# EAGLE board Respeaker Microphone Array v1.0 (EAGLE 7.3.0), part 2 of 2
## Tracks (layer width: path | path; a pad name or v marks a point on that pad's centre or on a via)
24MHZ  (via drill 0.25 pad 0.51)
  Top 0.203: U1.125 30.04,56.79 v29.96,56.87
  Top 0.305: v29.96,56.88 v29.96,56.87 30.15,57.07 R1.2
  Bottom 0.305: 24M.T 29.33,57.5 v29.96,56.87
24MHZ_8960  (via drill 0.25 pad 0.51)
  Top 0.254: U6.11 37.08,26.89 v37.07,26.9
  Top 0.406: R19.2 36.96,26.77 37.08,26.89
  Bottom 0.406: v37.07,26.9 37.07,27.28 24M_1.T
$123  (via drill 0.25 pad 0.51)
  Top 0.254: U6.29 43.6,26.39 v43.67,26.45
  Top 0.406: C90.1 49.51,21.82 48.5,22.83 v48.5,22.96
  Bottom 0.406: v43.67,26.45 43.8,26.58 44.43,26.58 44.94,26.07 44.94,24.1 46.08,22.96 v48.5,22.96
$124  (via drill 0.25 pad 0.51)
  Top 0.254: U6.31 43.63,27.39 v43.67,27.34
  Top 0.406: C91.1 47.86,21.82 | C91.1 47.48,21.82 | 46.47,21.69 46.59,21.56 46.97,21.56 47.1,21.69 C91.1 | v47.86,23.6 47.86,22.58 C91.1
  Bottom 0.406: v43.67,27.34 43.8,27.22 44.88,27.22 45.58,26.52 45.58,24.36 46.34,23.6 v47.86,23.6
_I2S_BCLK  (via drill 0.25 pad 0.51)
  Top 0.152: U6.12 37.44,26.39 36.94,25.88 v36.69,25.88 | v20.81,49.89 C83.1 R33.1
  Bottom 0.152: v36.69,25.88 35.92,26.64 35.92,31.6 34.65,32.87 34.65,39.47 35.42,40.23 35.42,41.76 33.38,43.79 30.21,43.79 25.38,38.96 20.94,38.96 19.03,40.87 19.03,48.11 v20.81,49.89
_I2S_DAC_DATA  (via drill 0.25 pad 0.51)
  Top 0.152: U6.14 37.59,25.39 37.19,24.99 v35.8,24.99 | v18.02,45.44 C80.1 R41.1
  Bottom 0.152: v35.8,24.99 35.16,25.63 35.16,31.34 33.89,32.61 33.89,39.73 34.65,40.49 34.65,41.5 33.13,43.03 30.59,43.03 25.76,38.2 20.69,38.2 18.02,40.87 v18.02,45.44
_I2S_LRCK  (via drill 0.25 pad 0.51)
  Top 0.152: U6.13 37.58,25.89 37.07,25.37 36.31,25.37 v35.8,25.88 | v18.53,47.6 C82.1 R40.1
  Bottom 0.152: v35.8,25.88 35.54,26.14 35.54,31.47 34.27,32.74 34.27,39.6 35.04,40.36 35.04,41.63 33.26,43.41 30.46,43.41 25.64,38.58 20.81,38.58 18.53,40.87 v18.53,47.6
AGND  (via drill 0.25 pad 0.51)
  Top 0.152: v39.48,27.03 v40.5,27.03 v41.51,27.03 | v39.48,25.25 v40.5,25.25 v41.51,25.25
  Top 0.203: SW1.3 43.58,16.07 43.29,16.36 v43.29,16.61 | SW1.7 44.36,14.33 44.43,14.26 44.62,14.26 | 44.62,14.26 45.13,14.26 v45.2,14.33 44.94,14.33 44.76,14.51 SW1.8 44.76,14.4 44.62,14.26
  Top 0.254: C4.1 44.54,26.37 44.06,25.89 U6.28 40.75,25.89 U6.33
  Top 0.305: R3.1 47.74,16.61 | 46.66,13.75 46.72,13.69 | D2.2 42.21,14 42.02,13.82 | D1.2 43.09,16.81 v43.29,16.61
  Top 0.356: R3.1 46.74,16.59 46.72,16.61 C92.1 46.72,16.76 45.12,18.37 C79.1
  Top 0.406: C89.1 45.55,27.56 v45.7,27.41
  Top 0.508: C89.1 45.55,28.45 | C71.1 45.7,29.18 | 45.58,32.61 U7.1 44.05,32.36 v43.93,32.49 | J9.5 37.09,0.97 36.81,1.24 36.81,1.75 | 36.81,1.75 R32.2 | J9.6 37.31,3.27 36.81,2.77 36.81,1.75
  Top 1.016: v50.07,28.76 48.45,28.76 v46.72,27.03 | 50.23,28.76 v50.07,28.76 | J3.14 v50.7,28.76 50.61,28.76 | 50.58,28.76 v50.07,28.76 | v50.07,28.76 50.02,28.8 | 50.61,28.76 50.58,28.76 | 50.58,28.76 49.89,29.44 | 50.61,28.76 50.02,28.17
  Bottom 1.016: J3.14 v50.07,28.76
  other vias: 40.24,0.99 44.05,2.01 44.05,5.18 46.72,12.93 42.53,13.44 42.53,17.37 46.59,26.14 40.5,26.14 39.48,26.14 41.51,26.14 40.12,29.95 41.39,29.95 44.43,11.28 40.37,7.72 43.42,6.96 40.75,5.18 38.08,2.13 38.21,9.63 38.21,15.98 38.21,17.37 39.48,17.37 40.75,17.37 46.47,11.28 45.45,11.28 42.4,32.49 44.81,30.84 44.81,29.31 38.85,2.13 39.61,2.13 43.54,8.74 41.64,10.01 43.67,10.01 42.53,11.53 44.05,12.55 41.64,13.06 48.37,30.84 49.64,30.84 49.64,31.85 48.37,31.85 41.39,31.22 38.21,14.71 38.21,13.44 38.21,12.17 48.24,26.01 48.37,29.31 48.37,12.93 49.01,14.33 50.91,14.33 48.37,11.66 46.59,6.58 46.72,3.91 49.18,26.03 47.35,26.01
  pour Top (isolate 0.254, rank 2): 45.7,-0.53 36.31,-0.53 36.31,4.17 37.07,4.93 37.19,16.98 37.18,18.18 arc-90 38.65,19.66 39.93,19.66 arc45 40.5,20.23 40.5,23.85 39.74,23.85 38.92,24.67 38.92,30.1 41.58,32.75 47.74,32.74 50.76,32.74 arc-90 52.31,31.19 52.31,28.8 52.32,24.8 52.31,24.61 52.31,24.49 52.31,13.44 52.32,13.45 52.31,13.06 52.31,11.15 arc-90 50.77,9.61 50.67,9.61 50.66,9.63 50.15,9.61 48.88,9.63 48.05,9.63 arc90 46.85,8.43 46.85,0.61
  pour PWR (isolate 0.254): 46.34,-0.53 37.96,-0.53 37.58,-0.15 37.58,16.96 38.11,17.5 49.95,17.5 52.31,15.14 52.31,12.8 47.71,10.9 47.59,10.9 46.85,10.16 46.85,-0.03
  pour PWR (isolate 0.254): 41.61,32.76 49.59,32.76 50.28,32.07 50.28,26.57 49.46,25.76 43.54,25.76 42.27,24.48 39.57,24.48 39.13,24.91 39.13,30.28
  pour Top (isolate 0.254, no thermals): 39.1,-0.03 36.69,-0.03 36.43,0.23 36.43,3.4 37.07,4.04 39.86,4.04 40.12,3.78 40.12,0.1 39.99,-0.03
AUX_SEL  (via drill 0.25 pad 0.51)
  Top 0.203: SW1.6 43.58,14.87 43.42,14.71 v43.42,13.56 R20.2 | J3.1 60.42,40.76 v60.44,40.74
  Bottom 0.203: v43.42,13.56 56.75,13.56 62.34,19.15 62.34,39.34 60.93,40.76 60.45,40.76 v60.44,40.74 60.42,40.76 J3.1
AVDD  (via drill 0.25 pad 0.51)
  Top 0.203: SW1.1 44.76,16.68 v44.94,16.87
  Top 0.254: U6.32 43.39,27.89 43.54,28.04 43.93,28.04
  Top 0.406: C89.2 v44.05,28.04 43.93,28.04 | U7.2 47.35,30.96 C68.2 C71.2 47.23,29.18 46.59,28.55 v46.34,28.55 | C79.2 45.07,16.99 v44.94,16.87 | R20.1 45.04,12.83 v45.07,12.8
  PWR 0.406: v45.07,12.8 44.56,13.31 44.56,16.48 v44.94,16.87 50.53,16.87 v52.82,19.15
  Bottom 0.406: v46.34,28.55 46.34,29.18 TP4.T | v46.34,28.55 45.83,28.55 | 45.83,28.55 44.56,28.55 v44.05,28.04 | v46.34,28.55 47.1,28.55 | 47.1,28.55 47.61,28.55 50.66,25.5 50.66,20.42 51.93,19.15 v52.82,19.15 | 45.83,28.55 46.47,29.18 | 47.1,28.55 46.59,29.06
CENTRAL_LED  (via drill 0.25 pad 0.51)
  Top 0.152: R34.2 33.52,31.09 v33.52,30.59 v33.51,30.58 | U1.32 33.15,41.78 v33.26,41.88 | J3.4 50.83,38.76 v50.28,38.2
  Top 0.305: J3.4 55.44,38.76 v55.48,38.71
  PWR 0.152: v33.51,30.58 33.64,30.45 38.46,30.45 41.39,33.38 45.45,33.38 v50.28,38.2
  Bottom 0.152: v33.51,30.58 33.51,39.85 34.27,40.61 34.27,41.38 33.77,41.88 v33.26,41.88
  Bottom 0.305: J3.4 55.44,38.76 v55.48,38.71
DEBUG_USBDM_N  (via drill 0.25 pad 0.51)
  Top 0.203: J1.2 27.56,6.04 27.69,6.17 27.69,6.83 27.23,7.3 D7.1 27.23,7.54 27.67,7.98 27.67,9.5 v27.54,9.63 27.67,9.75 27.67,10.52 28.18,11.02 31.86,11.02 32.24,11.4 32.24,12.29 31.99,12.55 31.59,12.55 R38.2
  Bottom 0.152: v27.54,9.63 DM.T
DEBUG_USBDP_P  (via drill 0.25 pad 0.51)
  Top 0.203: D8.1 28.49,7.54 | D8.1 28.49,7.49 28.05,7.92 28.05,9.37 v28.3,9.63 28.05,9.88 28.05,10.39 28.3,10.64 32.11,10.64 32.62,11.15 32.62,12.42 32.11,12.93 31.69,12.93 R4.2 | J1.3 28.21,5.99 28.05,6.15 28.05,6.81 28.49,7.25 D8.1
  Bottom 0.152: v28.3,9.63 DP.T
DOUT5  (via drill 0.25 pad 0.51)
  Top 0.152: SK7.3 51.45,10.16 47.99,6.71 v47.99,6.07 | SK6.1 34.79,7.08 v35.67,6.2
  Bottom 0.152: v35.67,6.2 36.05,5.82 47.74,5.82 v47.99,6.07
GND  (via drill 0.25 pad 0.51, 0.64 pad 1.27)
  Top 0.203: U1.104 38.44,54.81 v38.34,54.71
  Top 0.254: U6.20 40.25,22.43 C69.1 | U6.24 42.25,23.24 v42.53,22.96 | U6.9 37.73,27.89 37.58,28.04 v37.58,28.3 | U3.6 23.14,29.4 22.97,29.57
  Top 0.305: U3.6 24.86,29.4 U3.9 | U3.3 25.34,29.4 25.13,29.18 25.13,29.17 U3.9 | U2.6 22.08,21.57 U2.9 21.07,21.82 v20.94,21.69 | U2.3 22.08,22.07 v22.34,21.82 | U5.2 21.57,30.32 v21.51,30.26 | J1.5 29.51,6.01 29.7,6.2 v29.96,6.2 | D7.2 27.14,8.37 v26.91,8.61 | U10.4 34.41,17.59 v34.22,17.4 | MIC7.8 36.74,33.94 36.94,34.14 v37.19,34.14 | MIC7.2 34.37,34.74 34.58,34.96 MIC7.5 35.85,34.96 36.18,35.28 36.18,35.39 v36.17,35.41 | MIC7.7 36.11,32.56 36.31,32.36 v36.31,32.11 | v25.13,29.12 v25.13,29.13 U3.9 | 22.84,21.82 v22.34,21.82 | U2.1 23.08,21.93 v22.97,21.82 v22.34,21.82 | v33.89,57.38 33.89,57.44 34.65,58.2 v34.65,58.39 | v52.43,42.65 52.29,42.5 U11.4 52.29,40.98 52.18,40.87 | 22.46,37.95 22.33,37.81 U9.4 22.33,36.56 22.72,36.17 | MIC8.2 20.36,61.82 v20.43,61.89 | MIC9.2 3.05,34.64 v3.44,35.03 | MIC10.2 18.07,6.79 v18.07,7.04 | MIC11.2 49.82,5.74 v49.77,5.69 | MIC12.2 67.02,32.84 v66.66,32.49 | MIC13.2 51.93,60.76 v51.93,60.43 | MIC12.8 67.44,35.89 v67.42,35.92 | C109.1 67.1,36.42 v66.98,36.3 | C86.1 42.66,33.76 v42.91,34.01 43.01,33.91 C108.1 44.54,33.91 v44.56,33.88 | MIC10.8 20.35,4.84 20.94,5.44 v21.13,5.44 | MIC7.6 33.34,33.65 v32.94,33.25 | C103.1 33.41,9.9 v33.38,9.88 | U3.1 25.54,28.4 | 25.34,28.4 25.13,28.4 25.11,28.42 | 25.54,28.4 25.54,28.01 25.64,27.91 | 25.54,28.4 25.34,28.4 | 25.34,28.4 25.19,28.55 | v22.84,33.69 22.84,34.03 | 22.84,34.03 C87.1 22.74,34.29 22.84,34.39 | 22.84,34.39 23.35,34.9 | 22.84,34.03 22.84,34.39 | D8.2 28.49,8.41 28.69,8.61 v28.94,8.61
  Top 0.356: v25.32,34.52 27.14,34.52 C85.1
  Top 0.406: v25.13,30.71 25.11,30.69 U3.9 25.11,28.42 25.11,28.32 25.51,27.91 | C69.1 v39.48,22.2 | 18.76,7.11 v18.4,7.47 | 49.33,6.12 v49.26,6.2 | MIC7.2 33.43,34.18 33.38,34.14
  Top 0.508: C5.1 v27.41,38.7 v27.42,38.71 | R22.1 22.2,27.91 v21.95,27.66 | C31.1 39.84,58.37 v40.12,58.65 | C39.1 34.68,58.37 v34.65,58.39 | C52.1 36.92,58.37 v36.94,58.39 | C51.1 v37.96,59.02 v37.96,59.03 | R7.1 19.16,25.89 v19.03,26.01 | v28.18,58.14 28.9,58.14 C32.1 | C66.1 31.58,58.37 v31.61,58.39 | C26.1 32.22,58.37 v32.56,58.71 | X1.2 30.53,61.99 C24.1 | C75.1 33.87,57.4 v33.89,57.38 | C62.1 43.95,23.49 v43.93,23.47 | C74.1 45.8,59 v45.83,59.03 | C1.1 36.43,11.66 v36.31,11.53 | C107.1 35.29,27.91 v34.65,28.55 | C88.1 34.78,29.06 v34.65,29.18 | D9.- 36.82,31.09 v36.94,30.96 | X2.2 34.34,24.93 v34.15,24.74 34,24.59 C2.1 34,23.75 v34.02,23.72 | v26.65,27.53 26.65,26.77 27.14,26.29 C19.1 27.76,26.1 v27.8,26.14 | C64.1 17.7,33.12 v17.37,33.45 | v18.53,29.82 18.14,29.44 Q1.2 17.51,29.82 v17.26,29.82 | SK3.2 6.67,36.22 v6.59,36.3 | C57.1 5.53,29.97 v5.51,29.95 | C35.1 30.85,36.86 v31.16,36.55 | C42.1 31.87,36.62 v31.8,36.55 | C41.1 32.88,37 v32.43,36.55 | C34.1 30.82,37.08 30.84,37.06 | v23.73,44.04 24.11,43.66 C40.1 | C65.1 v16.74,55.22 v16.75,55.22 | C45.1 24.4,53.54 v23.99,53.95 | v23.48,42.84 23.48,42.37 C84.1 | C58.1 21.78,5.13 v21.7,5.05 | R32.1 35.82,2.43 v35.73,2.51 | R32.1 v35.1,1.75 | R32.1 35.82,1.2 v35.73,1.12 | v15.35,17.25 14.11,16 C14.1 13,13.5 v12.94,13.44 | C63.1 19.99,34.2 v19.92,34.26 | C85.1 27.9,34.8 28.5,34.2 v28.5,33.95 28.54,33.91 R11.1 | C20.1 24.34,33.86 25,34.52 v25.32,34.52 | C59.1 54.71,8.36 | 54.71,8.36 54.71,9.01 v54.47,9.25 | 54.71,8.36 54.73,8.33 C110.1 56.35,8.33 v56.37,8.36
  Top 0.61: v42.53,22.96 43.42,22.96 v43.93,23.47
  Bottom 0.305: v37.58,28.3 37.7,28.17 37.7,26.52 37.58,26.39
  other vias: 27.8,23.6 23.54,32.68 23.54,32.04 27.16,25.37 30.72,62.84 40.12,60.43 50.91,58.33 45.7,53.82 46.34,49.89 46.34,49 46.34,47.73 46.34,46.71 46.34,44.93 46.34,42.27 39.93,36.42 38.4,36.55 37.39,36.55 36.12,36.55 35.29,36.49 23.8,39.47 50.28,47.73 23.73,45.69 23.73,46.71 23.73,47.73 23.67,51.09 18.4,9.88 12.81,9.63 8.75,21.31 7.22,31.22 9.76,44.55 33.77,67.41 37.58,62.46 55.48,50.27 59.8,51.54 60.44,54.84 61.45,46.2 63.1,37.69 61.2,22.96 53.45,11.02 47.86,8.36 35.92,9.63 23.73,5.31 30.72,5.94 28.69,24.74 35.04,47.98 37.07,47.98 33,47.98 33,49.89 35.04,49.89 37.07,49.89 37.07,46.08 35.04,46.08 33,46.2 62.98,51.54 9,13.44 25.89,27.91 32.75,1.75 7.1,17.25 39.73,35.6 12.18,49.63 61.2,48.87 28.69,66.14 23.61,64.87 17,62.46 7.73,53.44 15.1,51.54 13.45,43.92 6.46,40.11 3.29,26.14 7.1,26.14 3.29,21.69 50.28,51.54 57.9,53.44 55.36,46.46 57.9,56.62 68.06,28.68 55.36,59.16 22.46,13.06 19.16,13.44 47.74,55.35 27.23,2.13 29.26,2.13 41.39,52.81 37.07,52.81 41.39,47.98 41.39,46.08 41.39,49.89 31.86,54.33 35.04,51.54 44.56,55.98 43.93,58.52 41.26,60.68 25.51,58.39 20.43,19.79 19.16,19.79 17.89,19.79 17.89,19.15 19.16,19.15 20.43,19.15 20.43,17.63 19.16,17.63 17.89,17.63 20.43,21.06 23.61,22.2 23.86,22.77 15.35,13.44 17.89,13.44 32.62,28.04 28.69,23.6 35.29,59.16 36.31,59.16 38.85,60.43 24.24,61.06 10.91,53.44 10.91,57.25 29.96,3.28 26.15,3.28 35.54,7.21 47.74,48.36 14.08,45.82 15.99,43.92 15.99,45.82 9,49.63 5.19,49.63 6.46,44.55 3.29,44.55 3.29,40.11 7.1,21.69 15.35,12.17 19.16,12.17 22.97,36.93 65.52,44.55 67.42,41.38 66.15,38.58 47.74,45.19 25.51,54.71 26.15,56.62 51.55,55.35 66.79,24.23 65.9,19.79 32.5,62.97 24.88,62.33 39.1,20.8 20.43,13.44 34.02,21.69 32.62,21.69 32.62,18.01 28.69,17.25 28.69,15.98 23.22,13.69 21.7,13.44 26.65,38.33 48.88,5.18 54.97,11.15 55.74,11.66 54.34,12.04 57.9,13.82 64.69,17.18 19.03,53.44 30.08,62.2 50.28,40.74 19.54,42.27 60.56,13.06 3.29,31.6 1.19,35.09 4.3,34.77 4.56,33.12 20.68,7.09 19.16,3.66 17.13,60.17 20.81,61 20.18,59.98 51.29,63.22 49.01,62.46 50.02,59.92 66.02,32.36 69.07,35.15 53.2,5.05 50.34,7.72 52.75,7.34 48.37,39.47 50.28,35.66 50.28,39.47 55.36,55.35 55.36,52.17 62.98,47.73 13.45,59.79 14.72,57.63 22.97,7.09 33.89,1.75 47.74,2.64 63.04,14.77 58.4,17.37 61.83,17.63 59.67,15.47 63.29,19.15 63.36,21.69 63.36,25.5 63.36,30.58 60.44,25.5 55.36,43.92 58.53,43.92 52.75,43.92 62.28,42.65 64.18,40.74 46.08,41.63 44.05,41.57 24.49,30.71 55.36,42.65 58.53,42.65 48.5,64.43 22.97,47.6 22.97,49.89 23.73,48.74 17.95,50.52 14.08,60.49 20.68,3.02 35.92,10.2 36.56,22.58 37.45,32.11 44.56,35.92 44.56,34.52 17,24.99 14.84,24.99 15.99,19.15 14.08,19.15 11.16,25.88 13.45,29.95 13.45,31.72 13.45,33.76 13.45,39.85 2.27,28.93 46.85,61.51 45.58,62.14 44.94,65.06 41.07,65.06 50.28,34.39 27.42,17.25 42.91,38.58 35.67,15.98 36.56,17.63 36.31,16.87 13.51,19.85 55.99,18.52 53.45,18.52 32.62,4.29 35.54,4.04 47.61,3.91 33.26,13.69 33,15.98 36.56,20.8 32.11,24.23 19.41,38.58 18.02,39.47 30.84,42.39 31.48,42.39
  pour Top (isolate 0.254, rank 6): -0.52,69.32 70.6,69.32 70.6,-0.53 -0.52,-0.53
  pour GND (isolate 0.254, rank 6, no thermals): -0.52,69.32 70.6,69.32 70.6,-0.53 2.02,-0.53 2.02,-1.17 -0.52,-1.17
  pour Bottom (isolate 0.254, rank 6): -0.52,69.32 70.6,69.32 70.6,-0.53 2.02,-0.53 2.02,-2.44 -0.52,-2.44
  pour PWR (isolate 0.254, no thermals): 32.5,50.52 37.58,50.52 37.58,45.44 32.5,45.44
  pour Top (isolate 0.254, rank 2, no thermals): 22.97,6.45 32.5,6.45 32.5,-1.17 22.97,-1.17
  pour Bottom (isolate 0.254, rank 2, no thermals): 22.97,6.45 30.64,6.45 31.1,5.99 31.1,4.67 32.5,3.52 32.5,-1.17 22.97,-1.17
HP_L  (via drill 0.25 pad 0.51)
  Top 0.203: SW1.4 43.17,15.67 v43.05,15.8
  Top 0.356: D1.1 42.47,15.91
  Top 0.406: J3.8 56.13,34.76 v56.24,34.65 | v43.05,15.8 42.93,15.91 D1.1 42.46,15.98 42.4,15.98 41.64,16.74 39.86,16.74 39.61,16.48 L4.1
  Bottom 0.406: J3.8 56.13,34.76 v56.24,34.65 56.24,25.76 58.4,23.6 58.4,19.53 54.67,15.8 v43.05,15.8
HP_R  (via drill 0.25 pad 0.51)
  Top 0.203: SW1.5 43.22,15.27 v43.04,15.09
  Top 0.406: J3.7 57.12,34.76 v57.01,34.65 | v43.04,15.09 42.85,14.9 D2.1 42.21,14.9 41.26,15.85 L3.1
  Bottom 0.406: J3.7 57.12,34.76 v57.01,34.65 57.01,26.01 59.04,23.98 59.04,19.28 54.85,15.09 v43.04,15.09
I2C_SCL  (via drill 0.25 pad 0.51)
  Top 0.152: R37.1 45.75,52.04 v46.21,52.04 46.24,52.07 R15.1 46.72,53.95 45.96,54.71 42.15,54.71 41.13,53.7 36.13,53.7 35.24,54.58 U1.112 | U6.17 38.75,23.5 37.96,22.71 v37.7,22.71
  Bottom 0.152: v46.21,52.04 45.07,50.9 45.07,32.61 42.53,30.07 42.53,24.36 42.15,23.98 38.97,23.98 v37.7,22.71
I2C_SDA  (via drill 0.25 pad 0.51)
  Top 0.152: R36.1 45.75,51.03 v46.21,51.03 46.24,51.06 R16.1 46.72,50.39 47.1,50.01 48.5,50.01 49.01,50.52 49.01,52.55 46.47,55.09 42.02,55.09 41,54.08 36.56,54.08 v36.31,54.33 | U1.113 34.84,54.14 v34.78,54.08 | U6.18 39.25,23.3 38.46,22.52 v38.46,22.07
  Bottom 0.152: v46.21,51.03 45.45,50.27 45.45,32.49 42.91,29.95 42.91,24.23 42.27,23.6 39.46,23.6 38.46,22.6 v38.46,22.07 | v36.31,54.33 35.04,54.33 v34.78,54.08
I2S_BCLK  (via drill 0.25 pad 0.51)
  Top 0.152: U1.15 28.08,48.58 v28.37,48.87 | R33.2 22.91,51.03 v22.97,51.09
  Bottom 0.152: v28.37,48.87 27.99,49.25 22.72,49.25 22.34,49.63 22.34,50.46 v22.97,51.09
I2S_DAC_DATA  (via drill 0.25 pad 0.51)
  Top 0.152: U1.21 29.3,46.18 v29.32,46.2 | R41.2 v22.97,46.46
  Bottom 0.152: v29.32,46.2 29.32,46.84 28.94,47.22 23.48,47.22 22.97,46.71 v22.97,46.46
I2S_LRCK  (via drill 0.25 pad 0.51)
  Top 0.152: U1.18 29.1,47.38 v29.32,47.6 | v22.97,48.74 R40.2
  Bottom 0.152: v29.32,47.6 28.69,48.23 23.48,48.23 v22.97,48.74
LED_DATA  (via drill 0.25 pad 0.51)
  Top 0.152: R44.1 38.82,63.83 v38.72,63.73 | SK0.3 34.17,62.18 v34.27,62.08
  Bottom 0.152: v38.72,63.73 35.92,63.73 v34.27,62.08
LED_DATA_IN  (via drill 0.25 pad 0.51)
  Top 0.152: R45.2 43.93,64.39 v43.93,65.13 43.8,65.25 42.02,65.25 41.77,65 U13.2 | R47.2 24.39,42.62 23.58,43.43 22.99,43.43 | C77.1 22.84,43.43 | 22.84,43.43 22.99,43.43 | 22.84,43.28 v22.84,43.03 22.46,43.41 | 22.84,43.28 22.84,43.43 | 22.99,43.43 22.84,43.28
  Top 0.254: 22.46,43.41 22.65,43.41 22.78,43.28
  PWR 0.152: v22.84,43.03 22.46,43.41 22.46,51.66 v24.88,54.08
  Bottom 0.152: v24.88,54.08 30.08,54.08 31.61,55.6 40.12,55.6 41.77,57.25 41.77,62.97 v43.93,65.13
MCLK  (via drill 0.25 pad 0.51)
  Top 0.152: U1.63 40.84,39.64 42.15,38.33 42.15,37.69 42.4,37.44 U8.2 v43.54,37.44 | R50.1 26.86,35.77 C85.2 30.49,35.77 v30.59,35.66
  PWR 0.152: v43.54,37.44 43.04,36.93 39.61,36.93 38.59,35.92 30.84,35.92 v30.59,35.66
MCLK_TILE1  (via drill 0.25 pad 0.51)
  Top 0.152: U1.20 28.56,46.58 v28.69,46.71 | C84.2 23.9,41.34 v23.92,41.31 24.11,41.5 R49.1
  Bottom 0.152: v28.69,46.71 28.05,46.08 28.05,45.82 29.13,44.74 29.13,44.49 28.88,44.23 28.62,44.23 27.29,45.57 27.03,45.57 26.78,45.31 26.78,45.06 28.11,43.73 28.11,43.47 27.86,43.22 27.61,43.22 26.15,44.68 25.89,44.68 25.51,44.3 25.26,44.3 25,44.55 24.75,44.55 24.49,44.3 24.49,44.11 24.88,43.73 24.88,43.41 24.62,43.15 24.62,42.9 25.95,41.57 25.95,41.31 25.7,41.06 25.45,41.06 25.19,41.31 v23.92,41.31
MIC_CLK
  Top 0.152: R42.1 42.37,34.88 C108.2 43.42,36.55 | 42.77,36.79 U8.1 43.42,36.79 | 43.42,36.79 43.66,36.79 | R48.2 44.34,36.79 43.72,36.79 43.66,36.79 | 43.42,36.55 43.42,36.79 | 43.42,36.55 43.29,36.68 | 43.66,36.79 43.42,36.55
MIC_CLK0  (via drill 0.25 pad 0.51)
  Top 0.152: MIC7.3 34.1,33.33 33,32.23 v33,32.11 | R29.2 21.32,42.29 C101.2 19.69,43.43 v19.54,43.28
  PWR 0.152: v33,32.11 33,32.36 32.88,32.49 26.53,32.49 21.57,37.44 21.57,38.2 21.32,38.46 20.68,38.46 20.56,38.58 20.56,38.96 20.68,39.09 22.65,39.09 22.78,39.22 22.78,39.6 22.65,39.73 21.57,39.73 21.45,39.85 21.45,40.23 21.57,40.36 22.65,40.36 22.78,40.49 22.78,40.87 22.65,41 21.57,41 19.54,43.03 v19.54,43.28
  Bottom 0.152: MIC_CLK0.T | MIC_CLK0.T 20.56,43.91 | MIC_CLK0.T 20.17,43.91 v19.54,43.28
MIC_CLK1  (via drill 0.25 pad 0.51)
  Top 0.152: MIC8.3 19.69,62.96 19.69,63.37 19.92,63.6 20.81,63.6 21.23,64.02 21.41,64.02 21.64,63.79 21.64,63.67 21.22,63.25 21.22,63.07 21.45,62.84 21.64,62.84 22.02,63.22 22.21,63.22 22.4,63.03 22.4,62.84 22.02,62.46 22.02,62.27 24.24,60.05 v24.24,56.62 | R26.2 22.4,42.33 v21.7,43.03 21.32,43.41 C94.2
  PWR 0.152: v21.7,43.03 21.7,54.08 v24.24,56.62
  Bottom 0.152: MIC_CLK1.T 22.34,43.66 v21.7,43.03
MIC_CLK2  (via drill 0.25 pad 0.51)
  Top 0.152: v3.92,36.3 2.27,36.3 1.66,35.69 1.66,35.23 2.2,34.69 MIC9.3 | v22.02,35.28 | R28.2 v22.01,35.28 v22.02,35.28 | C87.2 22.04,35.26 v22.02,35.28
  Bottom 0.152: v3.92,36.3 4.56,35.66 5.19,35.66 5.32,35.53 5.32,34.9 5.44,34.77 5.83,34.77 5.95,34.9 5.95,35.53 6.08,35.66 6.46,35.66 6.59,35.53 6.59,34.9 6.71,34.77 7.1,34.77 7.22,34.9 7.22,35.53 7.35,35.66 7.73,35.66 7.86,35.53 7.86,34.9 7.98,34.77 8.37,34.77 8.49,34.9 8.49,35.53 8.62,35.66 9,35.66 9.13,35.53 9.13,34.96 9.25,34.84 9.64,34.84 9.76,34.96 9.76,35.53 9.89,35.66 21.64,35.66 v22.02,35.28 MIC_CLK2.T
MIC_CLK3  (via drill 0.25 pad 0.51)
  Top 0.152: R30.2 v35.29,11.53 35.31,11.51 C104.2 | MIC10.3 16.9,5.66 16.62,5.94 v16.62,6.45
  Bottom 0.152: MIC_CLK3.T 36.94,9.88 v35.29,11.53 34.78,12.04 33.26,12.04 31.73,10.52 17.97,10.52 16.62,9.17 16.62,8.74 16.75,8.61 17.19,8.61 17.32,8.48 17.32,8.1 17.19,7.98 16.87,7.98 16.75,7.85 16.75,7.47 16.87,7.34 17.26,7.34 17.38,7.21 17.38,6.83 17.26,6.71 16.87,6.71 v16.62,6.45
MIC_CLK4  (via drill 0.25 pad 0.51)
  Top 0.152: R31.2 34.08,11.59 v34.02,11.53 34.08,11.47 C103.2 | MIC11.3 50.55,4.66 50.55,4.19 50.28,3.91 48.62,3.91 v47.86,4.67
  Bottom 0.152: v34.02,11.53 34.4,11.15 MIC_CLK4.T 34.4,7.98 34.27,7.85 32.94,7.85 32.81,7.72 32.81,7.34 32.94,7.21 34.21,7.21 34.34,7.09 34.34,6.71 34.21,6.58 32.94,6.58 32.81,6.45 32.81,6.07 32.94,5.94 34.21,5.94 34.34,5.82 34.34,5.44 34.21,5.31 33.07,5.31 32.94,5.18 32.94,4.86 33.13,4.67 v47.86,4.67
MIC_CLK5  (via drill 0.25 pad 0.51)
  Top 0.152: MIC12.3 67.87,32.8 68.56,32.11 v68.82,32.11 | R52.2 v51.41,47.72 v51.42,47.73 C106.2
  Bottom 0.152: v68.82,32.11 68.18,32.74 68.18,37.52 60.52,45.19 53.96,45.19 v51.42,47.73 50.54,48.6 MIC_CLK5.T
MIC_CLK6  (via drill 0.25 pad 0.51)
  Top 0.152: MIC13.3 53.39,61.88 v53.58,61.7 | R53.2 v52.56,47.72 v52.56,47.73 C105.2
  Bottom 0.152: v53.58,61.7 53.32,61.44 53.32,60.93 53.45,60.81 54.21,60.81 54.34,60.68 54.34,60.3 54.21,60.17 53.2,60.17 53.07,60.05 53.07,59.66 53.2,59.54 54.21,59.54 54.34,59.41 54.34,59.03 54.21,58.9 53.2,58.9 53.07,58.78 53.07,58.39 53.2,58.27 54.09,58.27 54.21,58.14 54.21,57.76 54.09,57.63 53.2,57.63 53.07,57.51 53.07,57.12 53.2,57 54.09,57 54.21,56.87 54.21,56.49 54.09,56.36 53.2,56.36 53.07,56.24 53.07,55.85 53.2,55.73 54.09,55.73 54.21,55.6 54.21,55.22 54.09,55.09 53.2,55.09 53.07,54.97 53.07,54.58 53.2,54.46 54.09,54.46 54.21,54.33 54.21,53.95 54.09,53.82 53.2,53.82 53.07,53.7 53.07,53.31 53.2,53.19 54.09,53.19 54.21,53.06 54.21,52.68 54.09,52.55 53.2,52.55 53.07,52.43 53.07,52.04 53.2,51.92 54.09,51.92 54.21,51.79 54.21,51.41 54.09,51.28 53.2,51.28 53.07,51.16 53.07,48.88 MIC_CLK6.T 52.56,48.34 v52.56,47.73
MIC_DATA0
  Top 0.152: MIC7.4 35.97,33.33 36.56,32.74 37.73,32.74 R65.2
MIC_DATA1
  Top 0.152: MIC8.4 16.75,61.88 15.82,60.95 R64.2
MIC_DATA2
  Top 0.152: MIC9.4 2.2,32.83 1.61,32.23 1.61,31.29 R62.1
MIC_DATA3
  Top 0.152: MIC10.4 19.54,4.65 19.54,4.19 19.82,3.91 20.43,3.91 20.63,4.11 R61.1
MIC_DATA4
  Top 0.152: MIC11.4 53.95,5.68 R60.1
MIC_DATA5
  Top 0.152: R58.1 68.06,36.86 68.44,36.48 68.44,35.28 67.87,34.71 MIC12.4
MIC_DATA6
  Top 0.152: MIC13.4 50.8,62.63 50.47,62.97 50.47,63.35 50.15,63.67 48.27,63.67 R63.2
N$1
  Top 0.152: U1.12 25.39,49.78 R14.1
N$2
  Top 0.152: R18.1 37.07,24.23 37.72,24.89 U6.15
N$3
  Top 0.305: U3.2 26.43,28.9 26.72,28.61
  pour Top (isolate 0.254, no thermals): 25.64,29.06 27.03,29.06 27.42,28.68 28.94,28.68 29.07,28.55 29.07,27.28 28.94,27.15 27.42,27.15 27.29,27.28 27.29,27.79 26.4,28.68 25.64,28.68 25.51,28.8 25.51,28.93
N$4
  Top 0.203: U1.48 34.84,38.25 R6.2
N$5
  Top 0.152: U1.10 26.59,50.58 25.38,51.79 R12.1
N$6
  Top 0.152: U1.27 26.66,43.78 25.76,44.68 R17.1
N$7  (via drill 0.25 pad 0.51)
  Top 0.152: R23.1 21.6,29.1 v21.64,29.06 21.67,29.1 R22.2 22.22,29.11 U5.3
  Bottom 0.152: v21.64,29.06 21.7,29.06 ADM_VIN.T
N$8  (via drill 0.25 pad 0.51)
  Top 0.305: U3.4 25.81,29.9 25.76,29.95 v25.76,30.26 | v27.8,31.98 27.52,32.26 R10.1 28.1,32.47 | R11.2 28.1,32.47 | 28.1,32.47 27.73,32.11
  Bottom 0.305: v25.76,30.26 26.08,30.26 v27.8,31.98
N$9
  Top 0.152: D11.- 18.86,29.27 Q1.3
N$10
  Top 0.152: 63.44,35.23 63.44,35.2 | 63.44,35.2 63.48,35.15 64.63,34.01 64.63,25.63 60.94,21.95 60.18,21.95 57.38,19.15 SK8.1 | SK9.3 63.41,35.23 63.44,35.2
N$11
  Top 0.305: X1.3 30.53,58.75 R1.1
N$12
  Top 0.152: R25.1 17.91,28.02 D11.+
N$13
  Top 0.152: SK2.3 9.95,46.64 10.78,47.47 13.19,47.47 14.08,48.36 14.08,53.42 17.15,56.49 19.41,56.49 20.56,57.63 20.67,57.63 20.68,57.63 SK1.1
N$14
  Top 0.305: U5.5 21.57,34.18 C63.2
N$15
  Top 0.152: U9.2 21.33,36.05 20.62,35.34 R28.1
N$16
  Top 0.152: U11.5 52.29,46 R53.1
N$17
  Top 0.152: SK2.1 12.08,47.85 9.51,47.85 7.48,45.82 7.48,33.12 6.67,32.31 SK3.3
N$18
  Top 0.203: SW1.2 44.36,16.56 44.18,16.74
  Top 0.508: C81.2 44.05,16.87 44.18,16.74
N$19
  Top 0.152: SK4.3 11.23,18.44 10.78,18.9 10.78,20.93 9.51,22.2 9.51,34.14 8.42,35.23 SK3.1
N$20
  Top 0.152: SK5.3 16.59,8.39 12.18,12.8 12.18,18.39 11.17,19.4 SK4.1
N$21
  Top 0.508: R19.1 34.35,26.77 X2.3
N$22
  Top 0.152: U9.5 22.33,41.3 R26.1
N$23
  Top 0.152: U10.5 34.41,13.44 R31.1
N$24
  Top 0.152: U9.7 R29.1
N$25
  Top 0.152: U12.2 25.13,41.27 R49.2
N$26
  Top 0.152: U12.7 25.13,35.56 R50.2
N$27  (via drill 0.25 pad 0.51)
  Top 0.406: v14.46,40.74 15.83,40.74 J2.1
  Bottom 0.406: J2.1 v14.48,40.76 v14.46,40.74
N$28
  Top 0.152: U10.7 35.41,13.24 R30.1
N$29
  Top 0.305: U2.2 22.58,23.21 22.72,23.34
  pour Top (isolate 0.254, no thermals): 22.4,22.2 22.72,22.2 22.78,22.26 22.78,23.03 23.99,24.23 23.99,25.69 23.8,25.88 22.91,25.88 22.78,25.76 22.78,24.17 22.34,23.72 22.34,22.26
N$30  (via drill 0.25 pad 0.51)
  Top 0.406: J2.2 v12.41,40.76 v12.43,40.74
  Bottom 0.406: v12.43,40.74 11.06,40.74 J2.2
N$31
  Top 0.152: U1.30 R47.1
N$32  (via drill 0.25 pad 0.51)
  Top 0.305: R5.1 18.04,25.48 19.01,24.51 R7.2 19.56,24.51 v19.67,24.61 | v21.19,22.45 21.39,22.45 U2.4
  Bottom 0.305: v19.67,24.61 19.67,23.98 v21.19,22.45
N$33
  Top 0.152: U11.7 51.29,46.14 R52.1
N$34  (via drill 0.25 pad 0.51)
  Top 0.406: v14.46,38.71 15.8,38.71 J2.3
  Bottom 0.406: J2.3 14.51,38.76 v14.46,38.71
N$35  (via drill 0.25 pad 0.51)
  Top 0.152: U1.71 48.36,44.18 v48.37,44.17 | R58.2 68.06,37.87 67.12,37.87 C109.2 67.1,38.39 66.02,39.47 v64.63,39.47
  Bottom 0.152: v64.63,39.47 64.5,39.47 60.82,43.15 49.39,43.15 v48.37,44.17
N$36  (via drill 0.25 pad 0.51)
  Top 0.152: U1.70 47.36,43.78 v47.61,43.54 | R60.2 54.64,7.34 v55.17,7.34 55.19,7.36 C110.2
  Bottom 0.152: v47.61,43.54 49.01,42.14 61.2,42.14 64.37,38.96 64.37,17.76 55.42,8.8 55.36,8.74 55.17,8.55 v55.17,7.34
N$37  (via drill 0.25 pad 0.51)
  Top 0.152: U1.69 45.22,43.38 45.7,42.9 v47.1,42.9 | R61.2 22.26,3.64 v22.21,3.59 22.25,3.55 C111.2
  Bottom 0.152: v47.1,42.9 48.24,41.76 61.07,41.76 64,38.82 64,17.89 49.39,3.28 32.62,3.28 31.99,3.91 22.53,3.91 v22.21,3.59
N$38  (via drill 0.25 pad 0.51)
  Top 0.152: U1.68 41.94,42.98 41,43.92 34.02,43.92 v32.62,42.52 | R62.2 3.29,30.58 v3.29,30.07 3.26,30.05 C112.2
  Bottom 0.152: v32.62,42.52 32.5,42.52 27.8,37.82 3.79,37.82 2.4,36.42 2.4,30.96 v3.29,30.07
N$39
  cutout PWR (isolate 0.254): 37.27,66.87 32.54,66.87 32.54,64.81 37.27,64.81
  cutout GND (isolate 0.254): 33.01,66.87 32.55,66.87 32.54,64.81 37.27,64.81 37.27,66.87
N$40  (via drill 0.25 pad 0.51)
  Top 0.152: U1.59 39.24,41.14 v40.12,42.01 | v46.21,63.22 46.85,63.22 R63.1 46.88,64.35 C115.2
  Bottom 0.152: v40.12,42.01 42.78,44.68 42.78,61.19 44.81,63.22 v46.21,63.22
N$41  (via drill 0.25 pad 0.51)
  Top 0.152: U1.58 38.84,41.76 v38.59,42.01 | v16.49,59.54 R64.1 14.73,59.54 C114.2
  Bottom 0.152: v38.59,42.01 35.92,42.01 30.34,47.6 30.34,50.77 29.45,51.66 21.95,51.66 21.07,52.55 21.07,55.85 17.38,59.54 v16.49,59.54
N$42  (via drill 0.25 pad 0.51)
  Top 0.305: J6.6 57.85,36.76 v57.77,36.68
  Bottom 0.305: J6.6 57.85,36.76 v57.77,36.68
N$43
  Top 0.152: J1.4 28.86,6.21 R43.2
N$44  (via drill 0.25 pad 0.51)
  Top 0.152: v30.84,6.71 32.5,6.71 33,6.2 34.65,6.2 35.53,5.33 SK6.3 | SK5.1 20.34,11.24 21.07,10.52 v21.07,10.01
  Bottom 0.152: v30.84,6.71 24.37,6.71 v21.07,10.01
N$45  (via drill 0.25 pad 0.51)
  Top 0.152: SK7.1 49.12,10.4 v49.51,10.01 | SK8.3 60.48,15.38 v59.8,14.71
  Bottom 0.152: v49.51,10.01 55.48,10.01 59.8,14.33 v59.8,14.71
N$46
  Top 0.152: U1.88 44.6,50.98 R36.2
N$47
  Top 0.152: SK10.3 59.42,48.77 59.42,46.33 60.94,44.81 60.94,32.99 61.66,32.28 SK9.1
N$48
  Top 0.152: SK10.1 58.67,45.68 48.24,56.11 48.24,58.52 47.86,58.9 47.86,59.18 SK11.3
N$49  (via drill 0.25 pad 0.51)
  Top 0.152: SK1.3 19.37,57.84 v20.3,58.78 | SK0.1 36.62,60.5 33.7,63.41 33.64,63.47 32.88,64.24 v31.23,64.24
  Bottom 0.152: v20.3,58.78 25.76,64.24 v31.23,64.24
N$50
  Top 0.152: R34.1 D9.+
N$51  (via drill 0.25 pad 0.51)
  Top 0.406: J2.4 12.38,38.76 v12.43,38.71
  Bottom 0.406: v12.43,38.71 11.09,38.71 J2.4
N$52  (via drill 0.25 pad 0.51)
  Top 0.305: J2.5 14.51,36.76 v14.46,36.8
  Bottom 0.305: J2.5 14.51,36.76 v14.46,36.8
N$53
  Top 0.152: U1.89 43.98,51.38 R37.2
N$54
  Top 0.406: J10.2 58.27,10.53 C98.2 56.9,11.97 C97.2 56.15,12.65 C95.2 54.68,14.12 L7.2
N$55
  Top 0.406: 45.47,7.87 45.58,7.98 | 45.07,7.98 45.32,7.98 45.45,7.85 | L3.2 40.75,13.94 40.75,8.41 41.56,7.59 45.2,7.59 45.45,7.85 | J9.3 45.47,7.87 | 45.47,7.87 45.45,7.85
N$56
  Top 0.203: SW1.9 45.87,14.87
  Top 0.406: 46.68,14.65 C93.2 | C93.2 R39.2 48.22,14.68 49.26,15.72 49.26,17.75 50.02,18.52 C90.2 | C93.2 46.53,14.87 45.87,14.87
N$57
  Top 0.406: J9.4 38.79,8.23 39.61,9.05 L4.2
N$58  (via drill 0.25 pad 0.51)
  Top 0.305: J2.6 12.38,36.76 v12.43,36.8
  Bottom 0.305: J2.6 12.38,36.76 v12.43,36.8
N$59  (via drill 0.25 pad 0.51)
  Top 0.305: J2.7 14.48,34.76 v14.46,34.77
  Bottom 0.305: J2.7 14.48,34.76 v14.46,34.77
N$60  (via drill 0.25 pad 0.51)
  Top 0.305: J2.8 12.41,34.76 v12.43,34.77
  Bottom 0.305: J2.8 12.41,34.76 v12.43,34.77
N$61
  Top 0.203: SW1.11 45.94,15.67 45.96,15.65
  Top 0.406: 45.89,15.65 45.96,15.65 46.68,15.65 C92.2 R3.2 48.27,15.62 48.62,15.98 48.62,17.37 47.48,18.52 C91.2
N$62  (via drill 0.25 pad 0.51)
  Top 0.254: U6.22 41.25,23.23 v41.64,22.83
  Top 0.406: L6.1 54.04,16.28 v53.32,16.99
  Bottom 0.406: v53.32,16.99 53.2,17.12 47.23,17.12 41.64,22.71 v41.64,22.83
N$63  (via drill 0.25 pad 0.51)
  Top 0.305: J2.9 14.48,32.76 v14.46,32.74
  Bottom 0.305: J2.9 14.48,32.76 v14.46,32.74
N$64  (via drill 0.25 pad 0.51)
  Top 0.305: J2.10 12.41,32.76 v12.43,32.74
  Bottom 0.305: J2.10 12.41,32.76 v12.43,32.74
N$65  (via drill 0.25 pad 0.51)
  Top 0.254: U6.19 39.75,23.1 v39.61,22.96
  Top 0.406: v52.69,16.48 53.32,15.85 53.32,15.21 53.31,15.2 L7.1
  Bottom 0.406: v39.61,22.96 40.37,22.96 46.85,16.48 v52.69,16.48
N$66
  Top 0.406: J10.1 58.77,11.54 C99.2 57.59,12.65 C97.1 56.9,13.4 56.18,14.13 C96.2 55.43,14.88 L6.2
N$67  (via drill 0.25 pad 0.51)
  Top 0.305: J2.11 14.51,30.76 v14.46,30.71
  Bottom 0.305: J2.11 14.51,30.76 v14.46,30.71
N$68  (via drill 0.25 pad 0.51)
  Top 0.305: J2.12 12.35,30.76 v12.43,30.84
  Bottom 0.305: J2.12 12.35,30.76 v12.43,30.84
N$69  (via drill 0.25 pad 0.51)
  Top 0.305: J2.14 12.38,28.76 v12.43,28.8
  Bottom 0.305: J2.14 12.38,28.76 v12.43,28.8
N$70  (via drill 0.25 pad 0.51)
  Top 0.305: J2.16 v12.41,26.76 v12.43,26.77
  Bottom 0.305: J2.16 v12.41,26.76 v12.43,26.77
N$71
  Top 0.152: U13.4 40,62.35 R44.2
N$72
  Top 0.152: R35.1 43.04,63.22 42.42,63.84 U13.1
N$73  (via drill 0.25 pad 0.51)
  Top 0.305: J3.6 55.4,36.76 v55.48,36.68
  Bottom 0.305: J3.6 55.4,36.76 v55.48,36.68
N$74  (via drill 0.25 pad 0.51)
  Top 0.305: J3.9 57.78,32.76 v57.77,32.74
  Bottom 0.305: J3.9 57.78,32.76 v57.77,32.74
N$75  (via drill 0.25 pad 0.51)
  Top 0.305: J3.10 55.47,32.76 v55.48,32.74
  Bottom 0.305: J3.10 55.47,32.76 v55.48,32.74
N$76  (via drill 0.25 pad 0.51)
  Top 0.305: J3.11 57.82,30.76 v57.77,30.71
  Bottom 0.305: J3.11 57.82,30.76 v57.77,30.71
N$77  (via drill 0.25 pad 0.51)
  Top 0.305: J3.12 55.4,30.76 v55.48,30.84
  Bottom 0.305: J3.12 55.4,30.76 v55.48,30.84
N$78  (via drill 0.25 pad 0.51)
  Top 0.305: J3.13 57.85,28.76 v57.77,28.68
  Bottom 0.305: J3.13 57.85,28.76 v57.77,28.68
N$79  (via drill 0.25 pad 0.51)
  Top 0.305: J3.16 55.47,26.76 v55.48,26.77
  Bottom 0.305: J3.16 55.47,26.76 v55.48,26.77
N$80
  Top 0.152: U8.4 41.12,38.09 41.77,37.44 41.77,35.21 R42.2 40.39,34.9 R46.2
N$81  (via drill 0.25 pad 0.51)
  Top 0.152: U1.62 40.44,39.27 v41,38.71 | R48.1 44.43,38.96 v43.93,39.47
  PWR 0.152: v43.93,39.47 41.77,39.47 v41,38.71
N$82  (via drill 0.25 pad 0.51)
  Top 0.152: U1.57 38.44,39.62 v38.85,39.22 | v39.1,33.76 39.08,33.74 R65.1 C113.2
  Bottom 0.152: v38.85,39.22 39.1,38.96 v39.1,33.76
N$83  (via drill 0.25 pad 0.51)
  Top 0.305: J6.4 57.82,38.76 v57.77,38.71
  Bottom 0.305: J6.4 57.82,38.76 v57.77,38.71
N$84
  cutout PWR (isolate 0.254): 47.1,38.2 49.51,38.2 49.51,37.69 47.1,37.69
N$85
  cutout PWR (isolate 0.254): 50.15,17.12 44.31,17.12 44.31,17.37 50.15,17.37
PG_3V3  (via drill 0.25 pad 0.51)
  Top 0.152: U3.5 23.65,29.9 v23.61,29.95 | R21.1 21,26.77 v20.24,27.53 19.92,27.85 19.92,29.06 20.92,30.05 U5.1
  Bottom 0.152: v23.61,29.95 23.61,27.91 22.84,27.15 20.56,27.15 | PG.T 20.43,27.28 | 20.43,27.28 20.43,27.35 v20.24,27.53 | 20.56,27.15 20.55,27.15 20.43,27.28 | 20.56,27.15 20.43,27.03
PLL_AVDD
  Top 0.203: U1.103 38.84,56.62 38.72,56.74
  Top 0.508: R13.1 41.03,59.43 C23.2 39.24,59.43 38.72,58.9 38.72,56.74
PLL_OUT  (via drill 0.25 pad 0.51)
  Top 0.152: 24.63,39.34 U12.6 24.63,35.04 v23.61,34.01 | 24.63,39.34 U12.3 | U12.1 25.63,39.34 25.51,39.22 24.76,39.22 | 24.76,39.22 24.63,39.34 | 24.76,39.22 24.75,39.22 24.65,39.12 | v34.91,24.23 R18.2 C78.2
  PWR 0.152: v34.91,24.23 34.91,27.53 31.35,31.09 26.53,31.09 v23.61,34.01
POR  (via drill 0.25 pad 0.51)
  Top 0.152: U5.4 22.22,32.37 v21.7,31.85 20.3,31.85 19.67,31.22 18.08,31.22 | R24.1 17.91,31.38 | 17.91,31.38 17.91,31.22 | 17.91,31.22 17.91,31.05 | 18.08,31.22 17.91,31.22 | 17.91,31.05 17.91,30.98 17.89,30.96 Q1.1 | 17.91,31.05 18.08,31.22 | 17.91,31.38 17.92,31.38 18.08,31.22 | U4.2 v17.38,49.12
  PWR 0.152: v21.7,31.85 21.7,33.38 17.38,37.69 v17.38,49.12
  Bottom 0.152: v21.7,31.85 21.96,31.85 POR.T
PRE_MIC_CLK  (via drill 0.25 pad 0.51)
  Top 0.152: U10.6 34.91,17.25 | 34.91,17.25 34.91,17.37 | 34.91,17.37 34.91,17.5 | 34.91,17.5 U10.3 | 35.04,17.37 34.91,17.37 | 34.91,17.5 35.04,17.37 | 34.91,17.25 35.04,17.37 | U11.1 50.79,42.51 | U11.3 51.79,42.47 | 51.79,42.47 51.79,42.65 | 51.79,42.65 51.79,42.83 | 50.79,42.53 50.79,42.64 50.78,42.65 | 51.61,42.65 51.79,42.65 | 51.79,42.83 51.61,42.65 | 51.79,42.47 51.61,42.65 | 35.04,17.37 35.67,17.37 35.91,17.62 U10.1 35.91,21.43 v35.92,21.44 | U11.6 51.79,42.83 | 51.61,42.65 50.91,42.65 | 50.91,42.65 50.78,42.65 | 50.78,42.65 50.66,42.65 | 50.79,42.51 50.66,42.65 | 50.79,42.51 50.79,42.53 | 50.79,42.53 50.91,42.65 | 50.66,42.65 v50.02,42.65 | v21.83,36.3 U9.3 21.83,36.93 | v21.83,36.3 | U9.6 21.83,37.69 | 21.83,37.69 21.83,36.93 | 21.83,36.93 | 21.7,37.69 21.07,37.69 20.83,37.46 U9.1 | 21.7,37.69 21.83,37.69 | 21.7,37.69 21.83,37.82 | 21.7,37.69 21.83,37.57 | C86.2 40.52,33.76 R46.1 v40.37,33.31
  PWR 0.152: v21.83,36.3 22.21,36.3 27.03,31.47 38.53,31.47 v40.37,33.31 42.21,35.15 44.81,35.15 46.59,36.93 46.59,39.85 49.39,42.65 v50.02,42.65
  Bottom 0.152: PMCK.T 41.39,32.36 41,31.98 39.86,31.98 39.48,32.36 39.23,32.36 38.97,32.11 38.97,31.85 39.48,31.34 39.48,31.09 39.1,30.71 38.85,30.71 38.15,31.41 37.89,31.41 37.64,31.15 37.64,30.9 38.34,30.2 38.34,29.82 38.08,29.57 38.08,24.87 35.92,22.71 35.54,22.71 35.42,22.58 35.42,22.2 35.54,22.07 35.8,22.07 35.92,21.95 v35.92,21.44 | PMCK.T | PMCK.T 40.55,33.13 v40.37,33.31
RST_N  (via drill 0.25 pad 0.51)
  Top 0.152: U4.4 18.03,52.3 | 18.03,52.3 18.03,52.41 | 18.03,52.41 18.03,52.67 v18.02,52.68 17.94,52.76 R27.1 | U1.123 v30.84,56.74 | U1.124 30.44,56.59 30.59,56.74 v30.84,56.74 | v27.92,56.24 27.29,55.6 24.88,55.6 21.57,52.3 18.27,52.3 | C66.2 31.17,57.07 v30.84,56.74 | 18.27,52.3 18.14,52.3 | 18.14,52.3 18.03,52.3 | 18.27,52.3 18.08,52.11 | 18.03,52.41 18.14,52.3
  Bottom 0.152: v27.92,56.24 30.34,56.24 v30.84,56.74 | RST.T 17.9,52.8 v18.02,52.68
SYS_1V  (via drill 0.25 pad 0.51)
  Top 0.203: U1.41 32.04,39.52 31.73,39.22 | U1.36 30.04,39.39 30.21,39.22 | U1.49 35.24,39.39 35.54,39.09 | U1.56 38.04,39.26 | U1.120 32.04,56.69 v31.99,56.74 | U1.126 29.64,56.42 29.32,56.74 29.26,56.74 v29.13,56.87 | U1.17 26.33,47.78 v26.27,47.73 26.73,48.18 U1.16 | U1.11 26.1,50.18 v25.76,50.52 | U1.24 26.22,44.98 v25.89,45.31 | U1.87 43.61,50.58 43.8,50.39 | U1.80 43.54,47.78 | 43.54,47.78 43.74,47.78 | 43.74,47.78 43.8,47.73 | U1.81 43.6,48.18 43.67,48.11 43.67,47.98 | 43.8,47.83 43.74,47.78 | 43.67,47.98 43.67,47.91 43.54,47.78 | 43.67,47.98 43.86,47.79 | U1.73 43.88,44.98 v43.93,44.93 | U1.60 39.64,39.31 39.73,39.22 | U1.101 39.64,56.58 39.61,56.62 39.48,56.62 39.35,56.49 | U1.102 39.24,56.38 39.35,56.49 | 39.35,56.49 39.48,56.49 39.61,56.36
  Top 0.508: 30.46,39.22 30.84,39.22 | 30.84,39.22 31.23,39.22 | 30.85,39.21 30.84,39.22 | C34.2 C35.2 v30.85,38.58 v30.84,38.58 30.84,38.84 | 30.84,39.22 30.84,38.84 | 30.21,39.22 30.46,39.22 | 30.46,39.22 30.84,38.84 | 31.73,39.22 31.23,39.22 | 31.23,39.22 30.84,38.84 | 35.54,39.09 36.06,38.58 v36.18,38.58 | C36.2 v36.18,38.58 | v36.18,38.58 | C37.2 v38.47,38.58 v38.46,38.58 38.04,39.01 38.04,39.26 | v31.99,56.75 v31.99,56.74 32.18,56.94 C26.2 | C28.2 v26.27,47.73 | C29.2 25.51,50.77 v25.76,50.52 | C33.2 25.51,45.69 v25.89,45.31 | C27.2 v44.18,50.01 43.8,50.39 | C30.2 v44.18,47.73 43.8,47.73 | C25.2 v43.93,44.93 | C38.2 v39.74,38.58 v39.73,38.58 39.73,39.22 | 39.61,56.62 39.61,57.28 | 39.61,57.28 C31.2 | 39.61,57.28 40.66,57.28 R13.2 v42.27,57.76 | C32.2 v29.14,56.88 v29.13,56.87 | R23.2 20.6,28.13 v20.43,28.3
  Bottom 0.508: v26.53,33.38 26.36,33.21 1V.T 23.62,31.09 21.19,31.09 20.43,30.33 v20.43,28.3
  other vias: 26.53,33.88 27.03,33.88 27.03,33.38 27.54,33.88
  pour Top (isolate 0.254, no thermals): 27.92,29.63 28.94,29.63 29.07,29.76 29.07,31.09 28.69,31.47 27.57,31.47 27.03,32.01 27.03,32.99 27.16,33.12 27.8,33.12 27.92,33.25 27.92,34.01 27.8,34.14 25.76,34.14 25.38,33.76 25.38,31.34 27.03,29.69 27.1,29.63
  pour PWR (isolate 0.254, rank 2, no thermals): 27.54,33.12 26.4,33.12 26.15,33.38 26.15,35.15 28.05,37.06 28.05,41.88 25.64,44.3 25.64,45.57 25.76,45.69 26.53,45.69 26.78,45.95 26.78,46.96 26.53,47.22 26.02,47.22 25.89,47.35 25.89,47.98 26.15,48.23 28.43,48.23 28.94,48.74 28.94,49.98 28.66,50.27 25.51,50.27 25.38,50.39 25.38,51.54 25.64,51.79 28.43,54.58 28.43,56.87 28.69,57.12 29.32,57.12 30.08,56.36 31.23,56.36 31.86,57 32.62,57 33.51,56.11 39.73,56.11 41.64,58.01 42.78,58.01 43.29,57.51 43.29,51.54 44.56,50.27 44.56,49.76 44.31,49.5 43.54,49.5 43.29,49.25 43.29,48.49 43.67,48.11 44.31,48.11 44.56,47.85 44.56,47.47 44.31,47.22 43.54,47.22 43.16,46.84 43.16,45.82 43.54,45.44 44.18,45.44 44.43,45.19 44.43,43.92 43.16,42.65 43.16,41 40.5,38.33 38.24,38.33 37.96,38.61 37.96,39.04 37.78,39.22 36.81,39.22 36.56,38.96 36.56,38.46 36.31,38.2 35.54,38.2 35.16,38.58 35.16,39.34 34.91,39.6 31.73,39.6 31.48,39.34 31.48,37.57 27.8,33.88 27.8,33.38
SYS_3V3  (via drill 0.25 pad 0.51)
  Top 0.203: U1.44 33.24,39.33 33.21,39.29 | 33,39.09 33.07,39.15 33,39.22 | 32.88,38.96 32.75,38.96 32.44,39.27 32.44,39.53 | U1.42 32.44,39.53 | 32.44,39.53 32.75,39.22 | U1.52 36.44,39.59 36.81,39.22 | U1.19 26.42,46.98 26.27,46.84 | U1.6 26.26,52.18 26.02,52.43 | U1.14 26.38,48.98 26.27,48.87 | U1.29 26.45,42.98 26.27,43.15 | U1.83 43.91,48.98 v43.93,49 | U1.78 43.78,46.98 43.93,46.84 | U1.67 43.74,42.58 43.8,42.52 | U1.105 38.04,56.66 v37.96,56.74 | U1.110 36.04,56.5 | 36.04,56.54 36.04,56.73 36.11,56.81 | U1.111 35.64,56.46 | 35.64,56.46 35.64,56.71 35.67,56.74 | 35.64,56.46 35.42,56.68 | 35.64,56.46 | 35.64,56.46 35.8,56.62 | 36.04,56.5 35.92,56.62 | 36.04,56.5 36.04,56.54 | 36.04,56.54 36.31,56.81 | U1.92 43.83,52.58 43.93,52.68
  Top 0.229: 48.9,61.42 49.11,61.42 49.48,61.79 50.35,61.79 MIC13.1 | 18.14,59.54 18.17,59.56 18.17,60.88 18.43,61.14 MIC8.1 | MIC9.1 3.05,32.82 3.9,31.98 3.92,31.98 | MIC10.1 20.44,5.73 20.85,6.13 21.09,6.13 | MIC11.1 52.03,6.8 52.03,7.7 | MIC12.1 67.02,34.69 66.21,35.5
  Top 0.254: MIC7.1 35.97,34.18 36.69,34.9 37.07,34.9 | U6.10 37.47,27.39 37.19,27.66 | U6.8 38.75,28.9 38.59,29.06 38.21,29.06
  Top 0.305: U12.8 25.63,37.18 25.76,37.31 26.53,37.31 v26.78,37.06 | U5.6 20.92,33.14 20.68,33.38 20.3,33.38 | U11.8 50.79,45.43 50.66,45.57 | U10.8 35.91,14.59 36.05,14.45 | U9.8 20.83,40.47 20.56,40.74
  Top 0.406: U4.5 16.73,53.45 C65.2 16.01,53.46 v15.99,53.44 | U8.5 41.2,36.49 v41.2,36.3 | C60.2 66.13,36.32 v66.15,36.3 66.15,35.56 66.21,35.5
  Top 0.508: 33,39.09 32.88,38.96 | C42.2 32.85,38.05 32.88,38.07 | 32.88,38.07 C41.2 | 32.88,38.07 v32.88,38.58 32.88,38.96 | 33.21,39.29 33.07,39.15 32.69,39.15 32.88,38.96 | C46.2 v37.33,38.58 v37.32,38.58 37.32,38.71 36.81,39.22 | C43.2 v26.02,46.71 26.15,46.71 26.27,46.84 | v25.38,53.44 25.37,53.42 C45.2 25.64,52.81 26.02,52.43 | C44.2 v25.89,48.74 26.15,48.74 26.27,48.87 | C40.2 25.76,43.66 v26.02,43.41 26.27,43.15 | C49.2 v43.93,49 | C48.2 v44.18,46.71 44.05,46.84 43.93,46.84 | 43.8,42.52 v44.18,42.52 44.43,42.52 44.69,42.27 C47.2 | C51.2 v37.96,56.75 v37.96,56.74 | 36.05,56.74 36.11,56.81 36.31,57 C52.2 36.92,57.4 v36.94,57.38 | C39.2 35.29,56.99 35.54,56.74 35.67,56.74 36.03,56.74 36.04,56.73 | C39.2 34.68,57.4 v34.65,57.38 | C39.2 36.28,57.4 36.31,57.38 | 43.93,52.68 44.05,52.81 v44.05,53.19 C50.2 | v47.74,52.68 47.69,52.64 R15.2 R16.2 | R2.2 v16.75,46.46 | C5.2 26.8,37.08 v26.78,37.06 | 37.07,34.9 38.08,34.9 | 38.08,34.9 C55.2 | 38.08,34.9 v38.08,34.26 | 20.3,33.38 19.67,33.38 v19.41,33.12 C64.2 | R24.2 v19.41,31.98 | R21.2 22.05,26.04 v22.08,26.01 | C67.2 | C67.2 50.17,46.22 49.99,46.04 | 49.99,46.04 49.77,45.82 v49.77,45.44 | 50.66,45.57 50.66,45.84 50.45,46.04 | 50.45,46.04 C67.2 | 36.05,14.45 36.43,14.07 v36.43,13.82 C1.2 | v31.73,62.84 31.71,62.82 C24.2 32.18,61.73 X1.1 32.24,60.92 32.18,60.86 X1.4 | 37.19,27.66 36.94,27.91 C107.2 36.41,29.03 36.43,29.06 | 38.21,29.06 36.43,29.06 | 36.43,29.06 C88.2 36.41,29.67 v36.43,29.69 | v33,23.6 33.03,23.62 C2.2 32.69,24.57 X2.1 X2.4 | 50.45,46.04 49.99,46.04 | R25.2 18.88,26.99 v18.53,27.34 | C70.2 v20.18,40.75 v20.18,40.74 20.56,40.74 | v4.56,29.95 v4.56,29.96 C57.2 4.56,31.33 3.92,31.98
  Top 0.508: 18.14,59.54 17,58.39 v16.49,58.39 16.46,58.43 C56.2 | 48.9,61.42 47.89,61.42 v47.86,61.44 47.85,61.45 C61.2 | 52.03,7.7 52.66,8.33 C59.2 53.74,9.09 v53.58,9.25 | v23.73,44.81 24.27,44.81 R17.2 | R27.2 17.94,55.2 v17.95,55.22 | 21.09,6.13 21.64,6.13 v21.7,6.07 21.73,6.1 C58.2
  Bottom 0.508: 3V3.T 19.17,22.83 v18.78,23.22
  other vias: 18.27,23.22 18.27,23.72 18.78,23.72 17.76,23.72 17.76,23.22
  pour Top (isolate 0.254, no thermals): 21.83,23.72 21.83,25.7 21.65,25.88 20.43,25.88 20.18,25.63 20.18,24.39 19.73,23.94 18.92,23.94 18.27,24.59 18.27,24.74 18.14,24.87 17.56,24.87 17.38,24.69 17.38,22.25 17.56,22.07 20.18,22.07
  pour PWR (isolate 0.254, rank 6, no thermals): -0.52,69.32 70.6,69.32 70.6,-0.53 2.02,-0.53 2.02,-1.8 -0.52,-1.8
TCK  (via drill 0.25 pad 0.51)
  Top 0.152: U1.128 28.84,53.6 v28.81,53.57
  Bottom 0.152: v28.81,53.57 28.81,53.32 TCK.T
TDI  (via drill 0.25 pad 0.51)
  Top 0.152: U1.2 26.48,53.78 v26.15,53.44
  Bottom 0.152: TDI.T v26.15,53.44
TDO  (via drill 0.25 pad 0.51)
  Top 0.152: U1.1 v27.29,54.58
  Bottom 0.152: v27.29,54.58 27.29,54.84 TDO.T
TMS  (via drill 0.25 pad 0.51)
  Top 0.152: U1.127 29.24,54.92 v29.57,54.58
  Bottom 0.152: TMS.T 29.57,55.1 v29.57,54.58
USBDM  (via drill 0.25 pad 0.51)
  Top 0.203: R9.1 27.43,12.28 v27.42,12.29 | J2.15 15.37,26.76 v14.72,27.41
  Bottom 0.203: v27.42,12.29 27.67,12.55 28.05,12.55 28.56,13.06 28.56,14.33 27.42,15.47 12.18,15.47 11.03,16.61 11.03,23.22 13.95,26.14 13.95,27.41 14.14,27.6 14.52,27.6 v14.72,27.41 15.37,26.76 J2.15
USBDP  (via drill 0.25 pad 0.51)
  Top 0.203: R8.1 27.43,13.3 v27.42,13.31 | J2.13 15.3,28.76 v14.72,28.17
  Bottom 0.203: v27.42,13.31 27.67,13.06 28.05,13.06 28.18,13.18 28.18,14.07 27.16,15.09 12.05,15.09 10.65,16.48 10.65,23.34 13.57,26.26 13.57,27.6 13.95,27.98 14.52,27.98 v14.72,28.17 15.3,28.76 J2.13
VDD_5V  (via drill 0.25 pad 0.51)
  Top 0.203: U1.45 v33.64,41.12
  Top 0.254: U6.26 43.65,24.89 v43.8,24.74 | U6.21 40.75,22.97 40.88,22.83
  Top 0.305: U3.7 23.64,28.9 23.48,28.74 23.48,28.55 | 23.48,28.36 23.48,28.04 | U3.8 23.63,28.4 23.48,28.55 | 23.48,28.55 23.48,28.36 | 23.48,28.36 23.22,28.1 | U2.7 22.58,20.49 | 22.58,20.49 22.58,20.35 22.37,20.14 | U2.5 21.58,20.41 21.83,20.17 22.34,20.17 22.37,20.14 | 22.37,20.14 23.1,19.41 C6.2 | U2.8 23.08,20.47 22.97,20.36 22.71,20.36 22.58,20.49 | C76.2 43.95,62.16 44.92,63.13 R35.2
  Top 0.356: J1.1 26.91,6.77 26.27,7.4
  Top 0.406: C62.2 44.08,24.46 v43.8,24.74 | 40.88,22.83 40.98,22.73 C69.2 41.26,21.92 C100.1 v41.26,20.04 | 42.53,62.2 42.53,62.24 U13.5 | v50.91,37.44 C3.2 C17.2 47.23,35.15 U7.3
  Top 0.508: R43.1 30.8,8.4 v30.84,8.36 31.12,8.63 C16.2 35.9,8.63 v35.92,8.61 36.6,7.93 SK6.4 | C21.2 25.61,23.37 v25.64,23.34 | v7.98,29.95 7.95,29.98 C13.2 8.42,31.07 SK3.4 | 23.08,11.91 C15.2 | C15.2 22.49,12.07 v22.46,12.04 | v45.2,57.51 v45.19,57.51 C74.2 46.61,58.03 SK11.4 | v20.43,54.46 20.4,54.43 C11.2 19.73,55.54 SK1.4 | 33.51,58.65 33.51,58.5 33.38,58.37 | v57.13,51.03 57.11,51.01 C73.2 57.11,48.68 SK10.4 | v60.31,23.98 59.69,23.36 C54.2 58.96,22.23 SK8.4 | v61.71,37.95 62.11,37.55 C72.2 61.66,36.61 SK9.4 | v52.82,12.8 C53.2 50.67,12.08 SK7.4 | v10.78,43.28 10.76,43.3 C12.2 10.76,45.38 SK2.4 | v10.4,25.88 10.4,25.05 arc45 10.98,23.65 arc-45 12.75,19.38 SK4.4 13,18.78 C14.2 13.55,16.97 v13.83,17.25 | v43.93,61.57 43.95,61.59 C76.2 42.59,62.14 42.53,62.2 | C75.2 33.38,58.37 | 33.38,58.37 33.81,58.37 v33.83,58.39 | 33.51,58.65 33.26,58.39 | 33.51,58.65 33.77,58.39 | 33.51,58.65 33.51,60.37 SK0.4 | SK5.4 23.08,11.68 | 23.08,11.68 23.08,11.89 23.1,11.91 23.08,11.91 | 23.08,11.91 | 23.08,11.68 22.72,12.04 | C15.2 24.14,12.07 | 24.21,12.07 24.98,12.07 25,12.04 | 24.14,12.07 24.62,12.55 | 24.14,12.07 24.21,12.07 | 24.21,12.07 24.62,11.66
  Top 0.813: J3.2 55.72,40.76 v55.74,40.74
  PWR 0.406: v50.91,37.44 51.42,37.44 | 51.42,37.44 52.05,37.44 | 51.42,37.44 51.93,37.95 | 51.42,37.44 51.8,37.06 | 56.24,42.65 56.24,42.14 55.61,41.5 | 43.93,60.68 43.93,61.06 43.42,61.57
  PWR 0.508: v25.64,18.45 25.19,18.45 | 25.19,18.45 15.03,18.45 v13.83,17.25 | v56.24,40.23 56.75,40.23 | 56.75,40.23 59.42,40.23 v61.71,37.95 | 56.75,40.23 v56.24,40.74 | 25.19,18.45 25.64,18.9 | v56.24,41.25 56.24,42.65 56.24,50.65 | 56.24,50.65 56.24,51.03 | 56.24,51.03 56.24,51.41 | 56.24,51.41 56.24,52.68 51.42,57.51 45.58,57.51 | 45.58,57.51 v45.2,57.51 45.2,57.89 | v57.13,51.03 56.63,51.03 | 56.63,51.03 56.24,51.03 | 56.63,51.03 56.24,51.41 | 56.63,51.03 56.24,50.65 | 45.2,57.89 45.2,58.52 43.93,59.79 43.93,60.68 v43.93,61.57 43.42,61.57 36.56,61.57 33.83,58.84 v33.83,58.39 | 45.2,57.89 45.58,57.51 | 54.34,24.99 59.29,24.99 v60.31,23.98 60.31,18.01 55.1,12.8 v52.82,12.8 | 54.34,24.99 53.32,24.99 | 54.34,24.99 53.7,25.63 | v10.4,25.88 10.4,29.44 | 10.4,29.44 10.4,29.95 | 10.4,29.95 10.4,30.45 | 10.4,30.45 10.4,42.9 v10.78,43.28 | v7.98,29.95 9.89,29.95 | 9.89,29.95 10.4,29.95 | 9.89,29.95 10.4,30.45 | 9.89,29.95 10.4,29.44
  Bottom 0.508: v30.84,8.36 29.96,7.47 26.53,7.47 25.13,8.86 v25.13,9.63 GND1.T | v33.64,41.12 31.86,41.12 29.19,38.46 29.19,26.39 26.15,23.34 v25.64,23.34 | v10.78,43.28 10.78,49.42 15.82,54.46 v20.43,54.46
  Bottom 0.813: J3.2 55.72,40.76 v55.74,40.74
  other vias: 25.64,18.96 26.15,18.45 26.15,18.96 26.15,19.47 25.64,19.47 55.74,41.25 55.74,40.23
  pour Top (isolate 0.254, no thermals): 26.65,4.55 27.03,4.55 27.16,4.67 27.16,6.32 26.4,7.09 26.4,26.14 25.51,27.03 24.62,27.91 24.62,28.3 23.28,28.3 23.1,28.12 23.1,27.28 24.37,26.01 24.37,7.59 26.53,5.44 26.53,4.67
  pour Top (isolate 0.254, no thermals): 22.59,14.58 23.99,14.58 24.49,14.07 24.49,21.44 24.49,21.82 24.11,21.44 23.1,21.44 22.97,21.31 22.97,20.55 22.72,20.29 22.46,20.04 22.46,14.71
  pour PWR (isolate 0.254, no thermals): 41,20.29 25.51,20.29 25.38,20.17 25.38,18.26 25.51,18.14 47.08,18.14 54.09,25.14 54.09,39.47 54.34,39.73 56.27,39.73 56.63,40.08 56.63,41.4 56.27,41.76 53.2,41.76 51.55,40.11 51.55,27.15 49.39,24.99 43.54,24.99 43.16,24.61 43.16,22.45
  pour Top (isolate 0.254, no thermals): 53.58,41.63 56.24,41.63 56.5,41.38 56.5,39.98 56.37,39.85 53.32,39.85 53.2,39.98 53.2,41.5 53.32,41.63
VMID  (via drill 0.25 pad 0.51)
  Top 0.254: U6.27 44.55,25.39 C4.2
  Top 0.406: C4.2 45.04,25.4 C102.1 45.96,24.61 v46.72,25.37
  Bottom 0.406: v46.72,25.37 46.72,24.74 TP14.T
XL_DN0  (via drill 0.25 pad 0.51)
  Top 0.152: U1.9 28.1,50.98 v28.3,50.77
  Bottom 0.152: XL_DN0.T 27.29,50.77 v28.3,50.77
XL_DN1  (via drill 0.25 pad 0.51)
  Top 0.152: U1.8 28.97,51.38 v29.32,51.03
  Bottom 0.152: XL_DN1.T v29.32,51.03
XL_UP0  (via drill 0.25 pad 0.51)
  Top 0.152: R12.2 24.11,51.79 v23.73,52.17
  Bottom 0.152: XL_UP0.T 24.25,52.68 v23.73,52.17
XL_UP1  (via drill 0.25 pad 0.51)
  Top 0.152: R14.2 v23.67,49.76
  Bottom 0.152: XL_UP1.T 24.18,50.27 v23.67,49.76
XSYS_RST_N  (via drill 0.25 pad 0.51)
  Top 0.152: R2.1 v16.75,48.74 16.73,48.76 U4.1
  Bottom 0.152: v16.75,48.74 16.75,47.85 RST_N.T
  Bottom 0.508: RST_N.T 15.73,47.73 J7.1
XUSBDM_N  (via drill 0.25 pad 0.51)
  Top 0.203: U1.47 34.44,37.1 30.84,33.5 30.84,15.47 30.97,15.34 v31.04,15.34 | R9.2 29.82,12.28 v29.83,12.29 29.84,12.28 R38.1
  Bottom 0.203: v29.83,12.29 30.08,12.55 30.59,12.55 31.1,13.06 31.1,14.58 30.97,14.71 30.97,15.28 v31.04,15.34
XUSBDP_P  (via drill 0.25 pad 0.51)
  Top 0.203: U1.46 34.04,37.21 30.46,33.63 30.46,15.47 v30.34,15.34 | R4.1 29.84,13.3 v29.83,13.31 v29.82,13.3 R8.2
  Bottom 0.203: v29.83,13.31 29.83,13.18 30.08,12.93 30.46,12.93 30.72,13.18 30.72,14.45 30.46,14.71 30.46,15.21 v30.34,15.34

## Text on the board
Top: 1
GND: 2
PWR: 3
Bottom: 4
bNames: ReSpeaker Microphone Array | v1.0 09/29/2016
